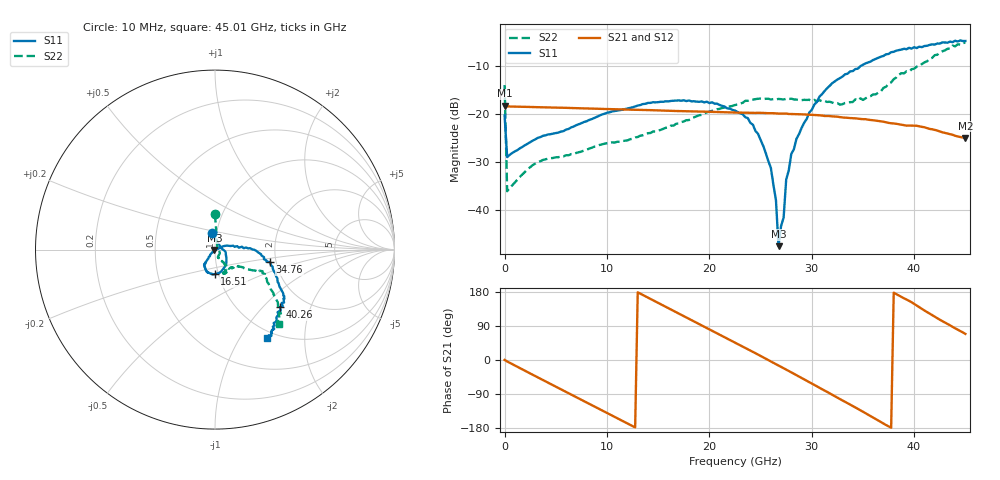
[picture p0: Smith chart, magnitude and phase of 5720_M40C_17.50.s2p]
! Device:  ADRF5720
! Description: 0.5dB LSB GaAs MMIC 6-bit Digital Attenuator
! Frequency:  0.000009 -  40 GHz
! Ports:
!	RF1	= Port 1
!	RF2	= Port 2
! Vdd:  3.3 Volt
! Vss:  -3.3 Volt
! Control:  0/3.3 Volt
! State:  17.50 dB attenuation
! Data:  The device was measured using G-S-G Probes on a matrix board.
!  Data was collected using an calibrated 4 port network analyzer.
!  The reference plane for this measurement is at the launchers.
! Note:  Analog Devices supplies this data as a sample of measured data
!  for this product.  Your particular data for this product may vary.
!  Data was taken at -40 degrees C.
!  Analog Devices reserves the right to change this data at anytime.
# GHZ S DB R 45.0
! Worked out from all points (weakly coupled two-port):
!   181 points, 10 MHz to 45.01 GHz, reference 45 ohm
!   highest |S21| = -18.27 dB at 10 MHz (marker M1); lowest = -25.0 dB at 45.01 GHz (marker M2)
!   lowest |S11| = -47.4 dB at 26.76 GHz (marker M3), VSWR 1.01, Z = 44.7 - j0.22 ohm
!   |S11| at or under -10 dB: start of sweep to 34.83 GHz
!   |S22| runs from -36.0 to -5.2 dB; largest |S21 - S12| = 0.00045
!   S11 on the Smith chart (normalised r, x): 10 MHz: 0.95, +0.18; 16.51 GHz: 0.96, -0.27; 34.76 GHz: 1.85, -0.29; 40.26 GHz: 1.51, -1.25; 45.01 GHz: 0.91, -1.32
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0.01  -20.32 101.6  -18.27 0.3  -18.29 0.2  -14.01 90.1
0.26  -28.97 14.8  -18.45 -3.8  -18.47 -3.9  -36.04 30.9
3.26  -24.97 -9.4  -18.60 -46.0  -18.63 -46.1  -29.95 -32.5
7.76  -21.68 -39.2  -18.85 -108.5  -18.87 -108.6  -27.60 -65.1
15.26  -17.48 -83.2  -19.28 147.1  -19.30 147.0  -23.31 -60.9
16.51  -17.27 -90.9  -19.38 129.7  -19.40 129.6  -22.43 -58.1
20.26  -17.59 -110.6  -19.58 77.3  -19.60 77.2  -19.38 -56.8
22.76  -19.60 -125.6  -19.72 42.4  -19.74 42.3  -18.05 -62.2
24.26  -22.24 -126.8  -19.79 21.5  -19.81 21.4  -17.04 -64.0
26.01  -31.17 -133.1  -19.85 -3.7  -19.87 -3.8  -17.01 -67.0
26.51  -37.91 -125.0  -19.89 -11.1  -19.91 -11.3  -17.02 -68.8
26.76  -47.44 -144.7  -19.93 -14.6  -19.95 -14.8  -16.89 -67.4
27.01  -43.27 -25.0  -19.93 -18.1  -19.95 -18.2  -16.94 -69.3
27.26  -41.48 35.5  -19.93 -21.8  -19.96 -21.9  -17.00 -68.2
27.51  -33.61 14.4  -19.93 -25.5  -19.95 -25.6  -16.87 -69.5
28.01  -28.29 19.5  -20.02 -32.6  -20.04 -32.8  -16.84 -70.5
30.26  -18.05 8.8  -20.22 -65.8  -20.24 -66.0  -17.09 -69.5
32.01  -13.62 0.3  -20.51 -91.8  -20.53 -91.9  -17.65 -62.0
34.76  -10.08 -12.8  -21.05 -132.8  -21.07 -132.9  -16.76 -44.6
37.76  -7.20 -31.6  -21.94 -178.7  -21.96 -178.9  -13.46 -31.0
40.26  -6.34 -41.4  -22.46 143.6  -22.47 143.4  -10.19 -26.0
45.01  -4.87 -59.2  -24.98 68.9  -25.00 68.8  -5.24 -49.4
